| TEXAS INSTRUMENTS INCORPORATED
| Standard Linear and Logic Group
| IBIS Model of SN74LVC827A
| 10-BIT BUFFER/DRIVER WITH 3-STATE OUTPUTS
| This file contains package information for the following:
|  SSOP 24-pin (DB) package as [Component] LVC827A_DB
|  TVSOP 24-pin (DGV) package as [Component] LVC827A_DGV
|  SOIC 24-pin (DW) package as [Component] LVC827A_DW
|  SOP 24-pin (NS) package as [Component] LVC827A_NS
|  TSSOP 24-pin (PW) package as [Component] LVC827A_PW
| This device can be powered at the following Vccs:
|  1.8 volt Vcc
|  2.5 volt Vcc
|  2.7 volt Vcc
|  3.3 volt Vcc
| This file provides unique models under the [Model Selector] for each Vcc.
| For operation at a specific Vcc, select the appropriate model after each
| [Model Selector] keyword.
[IBIS Ver]   3.2
[Comment char]  |_char
[File Name]   sn74lvc827a.ibs
[File Rev]   1.1 | a_die
[Date]   September 29, 2003
[Source]   Data created from TI-SPICE simulations at TI-SLL.
[Notes]   The following is an IBIS list for the LVC827A.
   Please contact sllibis@ti.com with questions and
   comments concerning SLL IBIS models.
   This IBIS model is created from a BA (back annotated netlist)
   - Due to the fact that the Device is 5-V Input/Output
   tolarent, the output model has some Non-Monotonic Warnings.
   - Power clamp data deleted as there is no power-clamp diode.
[Disclaimer] Property of Texas Instruments Incorporated.  Unauthorized
   reproduction and/or distribution is strictly prohibited.
   This product is protected under copyright law.
   Created  2003, (C) Copyright  2003, Texas Instruments
   Incorporated, All Rights Reserved
   UNLESS THERE IS A SIGNED, WRITTEN AGREEMENT TO THE
   CONTRARY, TEXAS INSTRUMENTS (TI) IS PROVIDING THE IBIS
   MODELS  AND WITHOUT ANY WARRANTY, EXPRESSED OR
   IMPLIED.  TI assumes no liability for:
   1) the accuracy of the IBIS models provided to your
   company;
   2) the proper functioning of these IBIS Models in your
   design or for any resulting applications; or
   3) infringement of patents, copyrights or intellectual
   property rights resulting from your use of these IBIS
   models.
   TI provides IBIS Models as a service to our customers.
   You and your company shall not distribute, sell or give
   these models to anyone else without prior written
   permission from TI.
   TI reserves the right to make changes to our products or
   to discontinue any semiconductor product or service
   without notice, and advises our customers to obtain the
   latest version of relevant information to verify, before
   placing orders, that the information being relied on is
   current.
   Please be aware that your receipt and use of the IBIS
   information provided shall serve as acceptance of these
   terms and conditions.  If you do not accept these terms,
   you should return or destroy the IBIS models and any
   other accompanying information immediately.
| Component LVC827A_DB 24-pin SSOP
[Component]   LVC827A_DB
[Manufacturer]   Texas Instruments, Inc.
[Package]
|   typ   min   max
R_pkg   4.500e-02   4.000e-02   4.900e-02
L_pkg   3.668e-09   3.226e-09   4.415e-09
C_pkg   4.160e-13   3.490e-13   5.070e-13
[Pin]   signal_name   model_name   R_pin   L_pin   C_pin
1   NOE1   LVC827A_NOE   4.200e-02   4.299e-09   5.030e-13
2   A1   LVC827A_IN   4.000e-02   3.960e-09   4.990e-13
3   A2   LVC827A_IN   4.200e-02   3.775e-09   4.170e-13
4   A3   LVC827A_IN   4.700e-02   3.487e-09   3.690e-13
5   A4   LVC827A_IN   4.600e-02   3.347e-09   3.520e-13
6   A5   LVC827A_IN   4.900e-02   3.352e-09   3.710e-13
7   A6   LVC827A_IN   4.600e-02   3.226e-09   3.630e-13
8   A7   LVC827A_IN   4.700e-02   3.289e-09   3.490e-13
9   A8   LVC827A_IN   4.700e-02   3.347e-09   3.610e-13
10   A9   LVC827A_IN   4.100e-02   3.576e-09   4.090e-13
11   A10   LVC827A_IN   4.100e-02   3.995e-09   5.030e-13
12   GND   GND   4.500e-02   4.415e-09   5.070e-13
13   NOE2   LVC827A_NOE   4.300e-02   4.337e-09   5.060e-13
14   Y10   LVC827A_OUT   4.200e-02   4.003e-09   5.040e-13
15   Y9   LVC827A_OUT   4.100e-02   3.686e-09   4.100e-13
16   Y8   LVC827A_OUT   4.800e-02   3.355e-09   3.490e-13
17   Y7   LVC827A_OUT   4.700e-02   3.301e-09   3.530e-13
18   Y6   LVC827A_OUT   4.800e-02   3.268e-09   3.660e-13
19   Y5   LVC827A_OUT   4.800e-02   3.269e-09   3.660e-13
20   Y4   LVC827A_OUT   4.700e-02   3.314e-09   3.490e-13
21   Y3   LVC827A_OUT   4.800e-02   3.399e-09   3.550e-13
22   Y2   LVC827A_OUT   4.100e-02   3.688e-09   4.120e-13
23   Y1   LVC827A_OUT   4.200e-02   4.003e-09   5.040e-13
24   VCC   POWER   4.300e-02   4.347e-09   5.050e-13
| Component LVC827A_DGV 24-pin TVSOP
[Component]   LVC827A_DGV
[Manufacturer]   Texas Instruments, Inc.
[Package]
|   typ   min   max
R_pkg   4.300e-02   3.900e-02   4.700e-02
L_pkg   2.601e-09   2.312e-09   3.626e-09
C_pkg   3.580e-13   2.770e-13   5.950e-13
[Pin]   signal_name   model_name   R_pin   L_pin   C_pin
1   NOE1   LVC827A_NOE   4.300e-02   3.625e-09   5.950e-13
2   A1   LVC827A_IN   4.000e-02   2.656e-09   4.020e-13
3   A2   LVC827A_IN   3.900e-02   2.338e-09   3.080e-13
4   A3   LVC827A_IN   4.600e-02   2.354e-09   2.770e-13
5   A4   LVC827A_IN   4.500e-02   2.312e-09   2.850e-13
6   A5   LVC827A_IN   4.700e-02   2.318e-09   2.820e-13
7   A6   LVC827A_IN   4.700e-02   2.318e-09   2.820e-13
8   A7   LVC827A_IN   4.500e-02   2.312e-09   2.850e-13
9   A8   LVC827A_IN   4.600e-02   2.353e-09   2.780e-13
10   A9   LVC827A_IN   3.900e-02   2.338e-09   3.080e-13
11   A10   LVC827A_IN   4.100e-02   2.660e-09   4.020e-13
12   GND   GND   4.300e-02   3.625e-09   5.950e-13
13   NOE2   LVC827A_NOE   4.400e-02   3.626e-09   5.940e-13
14   Y10   LVC827A_OUT   4.000e-02   2.658e-09   4.020e-13
15   Y9   LVC827A_OUT   3.900e-02   2.343e-09   3.110e-13
16   Y8   LVC827A_OUT   4.600e-02   2.353e-09   2.780e-13
17   Y7   LVC827A_OUT   4.500e-02   2.312e-09   2.850e-13
18   Y6   LVC827A_OUT   4.700e-02   2.319e-09   2.820e-13
19   Y5   LVC827A_OUT   4.700e-02   2.319e-09   2.820e-13
20   Y4   LVC827A_OUT   4.500e-02   2.312e-09   2.850e-13
21   Y3   LVC827A_OUT   4.600e-02   2.353e-09   2.780e-13
22   Y2   LVC827A_OUT   3.900e-02   2.337e-09   3.080e-13
23   Y1   LVC827A_OUT   4.000e-02   2.658e-09   4.020e-13
24   VCC   POWER   4.400e-02   3.626e-09   5.950e-13
| Component LVC827A_DW 24-pin SOIC
[Component]   LVC827A_DW
[Manufacturer]   Texas Instruments, Inc.
[Package]
|   typ   min   max
R_pkg   3.700e-02   3.000e-02   4.700e-02
L_pkg   5.146e-09   3.993e-09   6.885e-09
C_pkg   7.580e-13   5.120e-13   1.067e-12
[Pin]   signal_name   model_name   R_pin   L_pin   C_pin
1   NOE1   LVC827A_NOE   3.900e-02   6.885e-09   1.067e-12
2   A1   LVC827A_IN   4.200e-02   5.950e-09   9.580e-13
3   A2   LVC827A_IN   4.700e-02   5.317e-09   7.910e-13
4   A3   LVC827A_IN   3.100e-02   4.651e-09   6.110e-13
5   A4   LVC827A_IN   3.000e-02   3.993e-09   5.120e-13
6   A5   LVC827A_IN   3.000e-02   4.083e-09   6.110e-13
7   A6   LVC827A_IN   3.000e-02   4.083e-09   6.110e-13
8   A7   LVC827A_IN   3.000e-02   3.993e-09   5.120e-13
9   A8   LVC827A_IN   3.100e-02   4.652e-09   6.110e-13
10   A9   LVC827A_IN   4.700e-02   5.317e-09   7.910e-13
11   A10   LVC827A_IN   4.200e-02   5.950e-09   9.590e-13
12   GND   GND   3.900e-02   6.885e-09   1.067e-12
13   NOE2   LVC827A_NOE   3.900e-02   6.885e-09   1.067e-12
14   Y10   LVC827A_OUT   4.200e-02   5.950e-09   9.590e-13
15   Y9   LVC827A_OUT   4.700e-02   5.317e-09   7.910e-13
16   Y8   LVC827A_OUT   3.100e-02   4.652e-09   6.110e-13
17   Y7   LVC827A_OUT   3.000e-02   3.993e-09   5.120e-13
18   Y6   LVC827A_OUT   3.000e-02   4.083e-09   6.100e-13
19   Y5   LVC827A_OUT   3.000e-02   4.083e-09   6.100e-13
20   Y4   LVC827A_OUT   3.000e-02   3.993e-09   5.120e-13
21   Y3   LVC827A_OUT   3.100e-02   4.651e-09   6.110e-13
22   Y2   LVC827A_OUT   4.700e-02   5.317e-09   7.910e-13
23   Y1   LVC827A_OUT   4.200e-02   5.950e-09   9.580e-13
24   VCC   POWER   3.900e-02   6.885e-09   1.067e-12
| Component LVC827A_NS 24-pin SOP
[Component]   LVC827A_NS
[Manufacturer]   Texas Instruments, Inc.
[Package]
|   typ   min   max
R_pkg   4.400e-02   3.800e-02   4.800e-02
L_pkg   3.840e-09   2.545e-09   5.234e-09
C_pkg   5.860e-13   2.740e-13   7.970e-13
[Pin]   signal_name   model_name   R_pin   L_pin   C_pin
1   NOE1   LVC827A_NOE   4.100e-02   5.146e-09   7.650e-13
2   A1   LVC827A_IN   4.100e-02   4.357e-09   7.490e-13
3   A2   LVC827A_IN   4.000e-02   3.923e-09   6.330e-13
4   A3   LVC827A_IN   4.400e-02   3.412e-09   5.370e-13
5   A4   LVC827A_IN   4.500e-02   3.036e-09   3.970e-13
6   A5   LVC827A_IN   4.500e-02   2.845e-09   4.150e-13
7   A6   LVC827A_IN   4.400e-02   2.843e-09   4.150e-13
8   A7   LVC827A_IN   4.500e-02   3.065e-09   3.990e-13
9   A8   LVC827A_IN   4.500e-02   3.529e-09   5.440e-13
10   A9   LVC827A_IN   4.100e-02   4.013e-09   6.390e-13
11   A10   LVC827A_IN   4.100e-02   4.358e-09   7.460e-13
12   GND   GND   4.400e-02   5.234e-09   7.670e-13
13   NOE2   LVC827A_NOE   3.900e-02   5.181e-09   7.650e-13
14   Y10   LVC827A_OUT   4.800e-02   4.582e-09   7.640e-13
15   Y9   LVC827A_OUT   4.100e-02   4.163e-09   6.550e-13
16   Y8   LVC827A_OUT   4.600e-02   3.613e-09   5.490e-13
17   Y7   LVC827A_OUT   4.700e-02   3.163e-09   4.060e-13
18   Y6   LVC827A_OUT   4.700e-02   2.963e-09   4.220e-13
19   Y5   LVC827A_OUT   4.700e-02   2.919e-09   4.190e-13
20   Y4   LVC827A_OUT   4.800e-02   3.087e-09   4.870e-13
21   Y3   LVC827A_OUT   4.600e-02   4.513e-09   7.600e-13
22   Y2   LVC827A_OUT   4.200e-02   4.505e-09   7.670e-13
23   Y1   LVC827A_OUT   4.200e-02   5.163e-09   7.970e-13
24   VCC   POWER   3.800e-02   2.545e-09   2.740e-13
| Component LVC827A_PW 24-pin TSSOP
[Component]   LVC827A_PW
[Manufacturer]   Texas Instruments, Inc.
[Package]
|   typ   min   max
R_pkg   3.900e-02   3.000e-02   4.600e-02
L_pkg   2.685e-09   2.367e-09   3.177e-09
C_pkg   3.200e-13   2.520e-13   4.340e-13
[Pin]   signal_name   model_name   R_pin   L_pin   C_pin
1   NOE1   LVC827A_NOE   3.700e-02   3.153e-09   4.340e-13
2   A1   LVC827A_IN   3.400e-02   2.629e-09   3.410e-13
3   A2   LVC827A_IN   3.200e-02   2.860e-09   3.470e-13
4   A3   LVC827A_IN   4.200e-02   2.741e-09   2.900e-13
5   A4   LVC827A_IN   4.600e-02   2.600e-09   2.620e-13
6   A5   LVC827A_IN   4.300e-02   2.414e-09   2.660e-13
7   A6   LVC827A_IN   4.200e-02   2.367e-09   2.620e-13
8   A7   LVC827A_IN   4.400e-02   2.461e-09   2.520e-13
9   A8   LVC827A_IN   4.200e-02   2.543e-09   2.740e-13
10   A9   LVC827A_IN   3.000e-02   2.616e-09   3.320e-13
11   A10   LVC827A_IN   3.700e-02   2.670e-09   3.460e-13
12   GND   GND   3.900e-02   3.177e-09   4.330e-13
13   NOE2   LVC827A_NOE   3.700e-02   3.111e-09   4.310e-13
14   Y10   LVC827A_OUT   3.700e-02   2.656e-09   3.450e-13
15   Y9   LVC827A_OUT   3.100e-02   2.739e-09   3.400e-13
16   Y8   LVC827A_OUT   4.200e-02   2.649e-09   2.820e-13
17   Y7   LVC827A_OUT   4.600e-02   2.532e-09   2.570e-13
18   Y6   LVC827A_OUT   4.400e-02   2.425e-09   2.660e-13
19   Y5   LVC827A_OUT   4.400e-02   2.425e-09   2.660e-13
20   Y4   LVC827A_OUT   4.600e-02   2.532e-09   2.570e-13
21   Y3   LVC827A_OUT   4.200e-02   2.648e-09   2.820e-13
22   Y2   LVC827A_OUT   3.100e-02   2.738e-09   3.390e-13
23   Y1   LVC827A_OUT   3.600e-02   2.653e-09   3.440e-13
24   VCC   POWER   3.700e-02   3.110e-09   4.310e-13
| Model LVC827A_NOE
[Model Selector]   LVC827A_NOE
LVC827A_NOE_18   1.8 volt Vcc
LVC827A_NOE_25   2.5 volt Vcc
LVC827A_NOE_27   2.7 volt Vcc
LVC827A_NOE_33   3.3 volt Vcc
| Model LVC827A_IN
[Model Selector]   LVC827A_IN
LVC827A_IN_18   1.8 volt Vcc
LVC827A_IN_25   2.5 volt Vcc
LVC827A_IN_27   2.7 volt Vcc
LVC827A_IN_33   3.3 volt Vcc
| Model LVC827A_OUT
[Model Selector]   LVC827A_OUT
LVC827A_OUT_18   1.8 volt Vcc
LVC827A_OUT_25   2.5 volt Vcc
LVC827A_OUT_27   2.7 volt Vcc
LVC827A_OUT_33   3.3 volt Vcc
| Models and submodels in the file (12): LVC827A_NOE_18 (Input), LVC827A_NOE_25 (Input), LVC827A_NOE_27 (Input), LVC827A_NOE_33 (Input), LVC827A_IN_18 (Input), LVC827A_IN_25 (Input), LVC827A_IN_27 (Input), LVC827A_IN_33 (Input), LVC827A_OUT_18 (3-state), LVC827A_OUT_25 (3-state), LVC827A_OUT_27 (3-state), LVC827A_OUT_33 (3-state)
